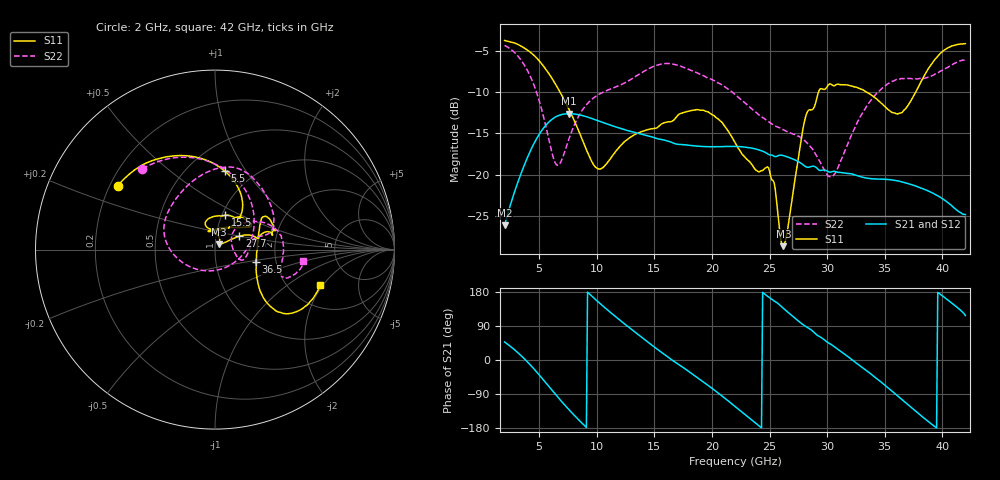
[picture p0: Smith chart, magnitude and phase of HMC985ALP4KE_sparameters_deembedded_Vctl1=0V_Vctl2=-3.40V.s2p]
!s2p File: Measurements: S11, S21, S12, S22
# GHz S dB R 50.0
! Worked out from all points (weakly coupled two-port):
!   401 points, 2 GHz to 42 GHz, reference 50 ohm
!   highest |S21| = -12.63 dB at 7.6 GHz (marker M1); lowest = -26.1 dB at 2 GHz (marker M2)
!   lowest |S11| = -28.6 dB at 26.2 GHz (marker M3), VSWR 1.08, Z = 52.3 + j3.02 ohm
!   |S11| at or under -10 dB: 6.804 GHz to 29.25 GHz (22.45 GHz wide, 125 % of centre); 33.41 GHz to 37.69 GHz (4.283 GHz wide, 12 % of centre)
!   |S22| runs from -20.3 to -4.4 dB; largest |S21 - S12| = 0.00049
!   S11 on the Smith chart (normalised r, x): 2 GHz: 0.23, +0.29; 5.5 GHz: 0.74, +0.81; 15.5 GHz: 1.04, +0.41; 27.7 GHz: 1.30, +0.20; 36.5 GHz: 1.57, -0.23; 42 GHz: 2.94, -1.89
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2  -3.77 146.6  -26.11 47.5  -26.11 47.5  -4.37 132.0
3.6  -4.60 119.5  -19.23 6.6  -19.24 6.6  -6.50 88.8
5.5  -7.11 82.9  -14.16 -57.3  -14.17 -57.3  -13.69 14.5
6.5  -9.25 65.6  -12.96 -93.6  -12.96 -93.6  -18.80 -63.1
7.6  -12.13 53.7  -12.63 -131.6  -12.63 -131.6  -15.62 -143.5
8.7  -15.62 54.2  -12.84 -166.1  -12.83 -166.2  -12.29 -177.3
10.3  -19.32 89.2  -13.57 148.6  -13.56 148.6  -10.20 157.2
12.6  -15.81 109.2  -14.64 90.8  -14.62 90.8  -8.78 123.8
15.4  -14.14 75.3  -15.70 25.3  -15.71 25.3  -6.69 83.2
15.5  -14.01 73.5  -15.72 23.1  -15.74 23.1  -6.66 82.1
19.3  -12.24 33.5  -16.60 -58.7  -16.60 -58.7  -8.05 37.8
22  -16.10 51.6  -16.58 -122.5  -16.59 -122.5  -10.31 16.3
24.9  -19.14 104.4  -17.54 166.5  -17.52 166.5  -13.58 11.1
26.2  -28.65 51.3  -17.70 136.4  -17.71 136.4  -14.57 -4.0
27.7  -16.19 28.8  -18.59 98.1  -18.60 98.0  -15.52 -19.7
28.7  -12.14 12.8  -18.98 77.3  -18.98 77.3  -16.85 -21.1
30.5  -9.22 18.4  -19.61 37.7  -19.62 37.8  -20.16 20.3
33.2  -9.83 34.3  -20.35 -23.3  -20.35 -23.3  -12.24 39.3
35.4  -12.23 11.7  -20.60 -76.3  -20.59 -76.3  -8.93 18.1
36.5  -12.49 -16.6  -20.88 -104.6  -20.89 -104.6  -8.38 6.6
39.5  -5.85 -43.6  -22.47 -179.2  -22.46 -179.3  -7.74 -21.9
42  -4.15 -18.7  -24.83 117.2  -24.82 117.1  -6.07 -7.5
